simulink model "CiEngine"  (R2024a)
settings: Solver=VariableStepAuto  StartTime=0.0  StopTime=inf  RelTol=1e-3  EnableMultiTasking=on
model workspace (MAT data in the model file):
  AccPwrTbl : Simulink.Parameter (value not decoded)
  AccSpdBpts : Simulink.Parameter (value not decoded)
  TimeCnstECP : Simulink.Parameter (value not decoded)
  TimeCnstEGR : Simulink.Parameter (value not decoded)
  TimeCnstETC : Simulink.Parameter (value not decoded)
  TimeCnstICP : Simulink.Parameter (value not decoded)
  TimeCnstIVL : Simulink.Parameter (value not decoded)
  TimeCnstSWVA : Simulink.Parameter (value not decoded)
  TimeCnstVCR : Simulink.Parameter (value not decoded)
  TimeCnstVGT : Simulink.Parameter (value not decoded)
  TimeCnstVIRL : Simulink.Parameter (value not decoded)
  TimeCnstWGA : Simulink.Parameter (value not decoded)
symbols that are objects in the model workspace (value not decoded): TimeCnstECP, TimeCnstEGR, TimeCnstETC, TimeCnstICP, TimeCnstIVL, TimeCnstSWVA, TimeCnstVCR, TimeCnstVGT, TimeCnstVIRL, TimeCnstWGA
libraries: autolibhevctrlrcommon x1, autolibpowerinfoutils x1, autolibutils x1

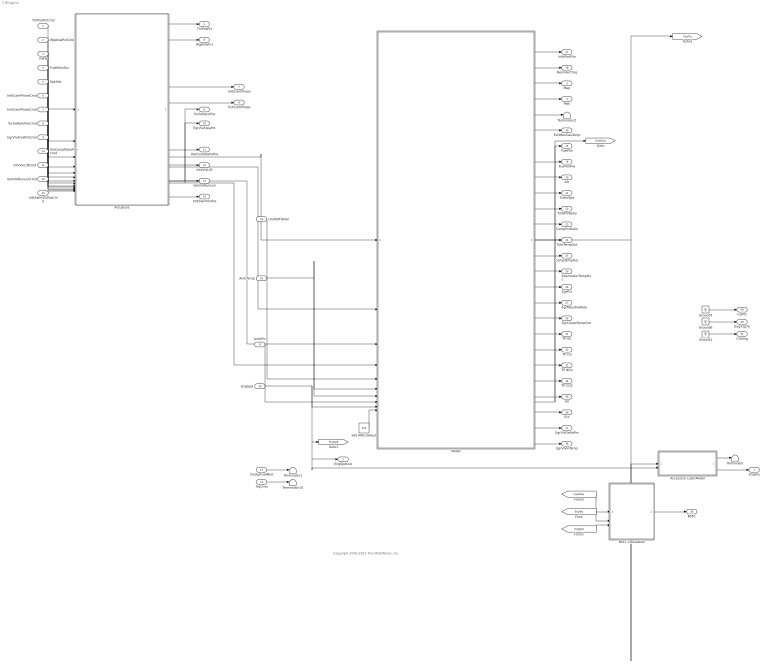
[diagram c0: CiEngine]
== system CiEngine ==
  note: Copyright 2020-2021 The MathWorks, Inc.
  ThrPosPctCmd : Inport
  WgAreaPctCmd : Inport  Port=2
  InjPw : Inport  Port=3
  FuelMainSoi : Inport  Port=4
  SpkAdv : Inport  Port=5
  IntkCamPhaseCmd : Inport  Port=6
  ExhCamPhaseCmd : Inport  Port=7
  TurboRackPosCmd : Inport  Port=8
  EgrVlvAreaPctCmd : Inport  Port=9
  VarCompRatioPosCmd : Inport  Port=10
  IntkVlvLiftCmd : Inport  Port=11
  VarIntkRunLenCmd : Inport  Port=12
  ClsdLpFuelMult : Inport  Port=13  Unit=1
  IntkSwirlVlvPosCmd : Inport  Port=14
  TrqCmd : Inport  Port=15  Unit=N*m
  AmbTemp : Inport  Port=16
  AmbPrs : Inport  Port=17
  EngSpd : Inport  Port=18  Interpolate=off
  UndHdFlwVel : Inport  Port=19
  100 MPa Default : Constant  Value=100
  Accessory Load Model : Subsystem
  Actuators : Subsystem
  BSFC Calculation : Subsystem
  Ground1 : Ground
  Ground5 : Ground
  Ground6 : Ground
  Model : ModelReference  ModelNameDialog=CiEngineCore  SimulationMode=Normal  ModelReferenceVersion=8.0
  Terminator{,1..2,15} (4 alike) : Terminator
  EngTrq : Outport  Unit=N*m  VectorParamsAs1DForOutWhenUnconnected=off
  EngSpdOut : Outport  Port=2  VectorParamsAs1DForOutWhenUnconnected=off
  Map : Outport  Port=3  VectorParamsAs1DForOutWhenUnconnected=off
  Mat : Outport  Port=4  VectorParamsAs1DForOutWhenUnconnected=off
  ThrPosPct : Outport  Port=5  VectorParamsAs1DForOutWhenUnconnected=off
  WgAreaPct : Outport  Port=6  VectorParamsAs1DForOutWhenUnconnected=off
  IntkCamPhase : Outport  Port=7  VectorParamsAs1DForOutWhenUnconnected=off
  ExhCamPhase : Outport  Port=8  VectorParamsAs1DForOutWhenUnconnected=off
  TurboRackPos : Outport  Port=9  VectorParamsAs1DForOutWhenUnconnected=off
  EgrVlvAreaPct : Outport  Port=10  VectorParamsAs1DForOutWhenUnconnected=off
  VarCompRatioPos : Outport  Port=11  VectorParamsAs1DForOutWhenUnconnected=off
  IntkVlvLift : Outport  Port=12  VectorParamsAs1DForOutWhenUnconnected=off
  VarIntkRunLen : Outport  Port=13  VectorParamsAs1DForOutWhenUnconnected=off
  IntkSwirlVlvPos : Outport  Port=14  VectorParamsAs1DForOutWhenUnconnected=off
  FuelFlw : Outport  Port=15  VectorParamsAs1DForOutWhenUnconnected=off
  FuelVolFlw : Outport  Port=16  VectorParamsAs1DForOutWhenUnconnected=off
  IntkPortFlw : Outport  Port=17  VectorParamsAs1DForOutWhenUnconnected=off
  NormAirChrg : Outport  Port=18  VectorParamsAs1DForOutWhenUnconnected=off
  ExhManGasTemp : Outport  Port=19  VectorParamsAs1DForOutWhenUnconnected=off
  Afr : Outport  Port=20  VectorParamsAs1DForOutWhenUnconnected=off
  TurboSpd : Outport  Port=21  VectorParamsAs1DForOutWhenUnconnected=off
  TurbPrsRatio : Outport  Port=22  VectorParamsAs1DForOutWhenUnconnected=off
  CompPrsRatio : Outport  Port=23  VectorParamsAs1DForOutWhenUnconnected=off
  TurbTempOut : Outport  Port=24  VectorParamsAs1DForOutWhenUnconnected=off
  CompTempOut : Outport  Port=25  VectorParamsAs1DForOutWhenUnconnected=off
  EgrPct : Outport  Port=26  VectorParamsAs1DForOutWhenUnconnected=off
  EgrMassFlwRate : Outport  Port=27  VectorParamsAs1DForOutWhenUnconnected=off
  EgrCoolerTempOut : Outport  Port=28  VectorParamsAs1DForOutWhenUnconnected=off
  IntercoolerTempOut : Outport  Port=29  VectorParamsAs1DForOutWhenUnconnected=off
  BSFC : Outport  Port=30  Unit=g/(kW*hr)  VectorParamsAs1DForOutWhenUnconnected=off
  TP HC : Outport  Port=31  VectorParamsAs1DForOutWhenUnconnected=off
  TP CO : Outport  Port=32  VectorParamsAs1DForOutWhenUnconnected=off
  TP NOx : Outport  Port=33  VectorParamsAs1DForOutWhenUnconnected=off
  TP CO2 : Outport  Port=34  VectorParamsAs1DForOutWhenUnconnected=off
  Iat : Outport  Port=35  VectorParamsAs1DForOutWhenUnconnected=off
  Ect : Outport  Port=36  VectorParamsAs1DForOutWhenUnconnected=off
  EgrVlvDeltaPrs : Outport  Port=37  VectorParamsAs1DForOutWhenUnconnected=off
  EgrVlvInTemp : Outport  Port=38  VectorParamsAs1DForOutWhenUnconnected=off
  CylPrs : Outport  Port=39  VectorParamsAs1DForOutWhenUnconnected=off
  EngTrqCrk : Outport  Port=40  VectorParamsAs1DForOutWhenUnconnected=off
  CrkAng : Outport  Port=41  VectorParamsAs1DForOutWhenUnconnected=off
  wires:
  EngSpd/1 -> Accessory Load Model/2(EngSpd), EngSpdOut/1, [EngSpd], Model/9
  Model/1 -> Accessory Load Model/1(EngTrqIn), [EngTrq]
  TrqCmd/1 -> Terminator15/1
  [FuelFlow] -> BSFC Calculation/1(FuelFlow)
  [EngTrq] -> BSFC Calculation/2(EngTrq)
  [EngSpd] -> BSFC Calculation/3(EngSpd)
  BSFC Calculation/1(BSFC (g/Kwh)) -> BSFC/1
  Model/8 -> FuelFlw/1, [FuelFlow]
  AmbTemp/1 -> Model/6, Model/7
  Actuators/1(ThrPosPct) -> ThrPosPct/1
  Actuators/2(WgAreaPct) -> WgAreaPct/1
  AmbPrs/1 -> Model/8
  UndHdFlwVel/1 -> Model/5
  Actuators/3(InjPw) -> Model/1
  Actuators/4(FuelMainSoi) -> Model/2
  Actuators/7(TurboRackPos) -> TurboRackPos/1, Model/3
  Actuators/8(EgrVlvAreaPct) -> EgrVlvAreaPct/1, Model/4
  Actuators/5(IntkCamPhase) -> IntkCamPhase/1
  Actuators/6(ExhCamPhase) -> ExhCamPhase/1
  Actuators/9(VarCompRatioPos) -> VarCompRatioPos/1
  Actuators/10(IntkVlvLift) -> IntkVlvLift/1
  Actuators/12(IntkSwirlVlvPos) -> IntkSwirlVlvPos/1
  Actuators/11(VarIntkRunLen) -> VarIntkRunLen/1
  ThrPosPctCmd/1 -> Actuators/1(ThrPosPctCmd)
  WgAreaPctCmd/1 -> Actuators/2(WgAreaPctCmd)
  InjPw/1 -> Actuators/3(InjPwCmd)
  FuelMainSoi/1 -> Actuators/4(FuelMainSoiCmd)
  SpkAdv/1 -> Actuators/5(SpkAdvCmd)
  IntkCamPhaseCmd/1 -> Actuators/6(IntkCamPhaseCmd)
  ExhCamPhaseCmd/1 -> Actuators/7(ExhCamPhaseCmd)
  TurboRackPosCmd/1 -> Actuators/8(TurboRackPosCmd)
  EgrVlvAreaPctCmd/1 -> Actuators/9(EgrVlvAreaPctCmd)
  VarCompRatioPosCmd/1 -> Actuators/10(VarCompRatioPosCmd)
  IntkVlvLiftCmd/1 -> Actuators/11(IntkVlvLiftCmd)
  VarIntkRunLenCmd/1 -> Actuators/12(VarIntkRunLenCmd)
  ClsdLpFuelMult/1 -> Terminator1/1
  IntkSwirlVlvPosCmd/1 -> Actuators/13(IntkSwirlVlvPosCmd)
  Model/2 -> IntkPortFlw/1
  Model/3 -> NormAirChrg/1
  Model/4 -> Map/1
  Model/5 -> Mat/1
  Model/7 -> ExhManGasTemp/1
  Model/6 -> Terminator2/1
  Model/10 -> Afr/1
  Model/11 -> TurboSpd/1
  Model/12 -> TurbPrsRatio/1
  Model/13 -> CompPrsRatio/1
  Model/14 -> TurbTempOut/1
  Model/15 -> CompTempOut/1
  Model/16 -> IntercoolerTempOut/1
  Model/17 -> EgrPct/1
  Model/18 -> EgrMassFlwRate/1
  Model/19 -> EgrCoolerTempOut/1
  Model/20 -> TP HC/1
  Model/21 -> TP CO/1
  Model/22 -> TP NOx/1
  Model/23 -> TP CO2/1
  Model/25 -> Ect/1
  Model/26 -> EgrVlvDeltaPrs/1
  Model/27 -> EgrVlvInTemp/1
  Model/24 -> Iat/1
  100 MPa Default/1 -> Model/10
  Accessory Load Model/2(EngTrqOut) -> EngTrq/1
  Accessory Load Model/1(PwrInfo) -> Terminator/1
  Model/9 -> FuelVolFlw/1
  Ground5/1 -> CylPrs/1
  Ground6/1 -> EngTrqCrk/1
  Ground1/1 -> CrkAng/1

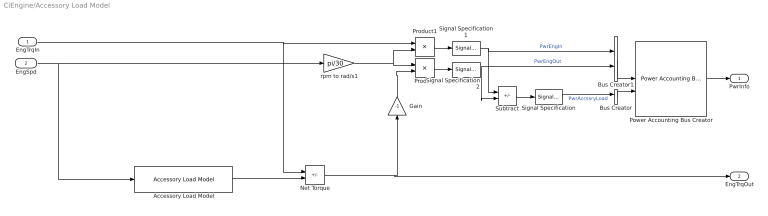
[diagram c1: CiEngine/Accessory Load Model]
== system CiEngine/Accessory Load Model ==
  EngTrqIn : Inport
  EngSpd : Inport  Port=2
  Accessory Load Model : autolibhevctrlrcommon/Accessory Load Model  AccPwrTbl=AccPwrTbl  AccSpdBpts=AccSpdBpts
  Bus Creator : BusCreator  Inputs=1
  Bus Creator1 : BusCreator  Inputs=2
  Gain : Gain  Gain=-1
  Net Torque : Sum  Inputs=+-
  Power Accounting Bus Creator : autolibpowerinfoutils/Power Accounting Bus Creator  AssctBlkSelPopup=Parent  RefBlkName='libraryname/blkname'  PwrTrnsfrdCheckBox=on  PwrNotTrnsfrdCheckBox=on  PwrStoredCheckBox=off  aMode=aMode
  Product : Product
  Product1 : Product
  Signal Specification : SignalSpecification  Unit=W
  Signal Specification1 : SignalSpecification  Unit=W
  Signal Specification2 : SignalSpecification  Unit=W
  Subtract : Sum  Inputs=--
  rpm to rad/s1 : Gain  Gain=pi/30
  PwrInfo : Outport  VectorParamsAs1DForOutWhenUnconnected=off
  EngTrqOut : Outport  Port=2  Unit=N*m  VectorParamsAs1DForOutWhenUnconnected=off
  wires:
  EngSpd/1 -> Accessory Load Model/1, rpm to rad/s1/1
  Net Torque/1 -> EngTrqOut/1, Gain/1
  Bus Creator/1 -> Power Accounting Bus Creator/2
  Bus Creator1/1 -> Power Accounting Bus Creator/1
  EngTrqIn/1 -> Product1/1, Net Torque/1
  Subtract/1 -> Signal Specification/1
  Signal Specification/1 -> Bus Creator/1  "PwrAccssryLoad"
  Power Accounting Bus Creator/1 -> PwrInfo/1
  Product/1 -> Signal Specification2/1
  Product1/1 -> Signal Specification1/1
  rpm to rad/s1/1 -> Product1/2, Product/1
  Signal Specification1/1 -> Subtract/1, Bus Creator1/1  "PwrEngIn"
  Signal Specification2/1 -> Subtract/2, Bus Creator1/2  "PwrEngOut"
  Gain/1 -> Product/2
  Accessory Load Model/1 -> Net Torque/2

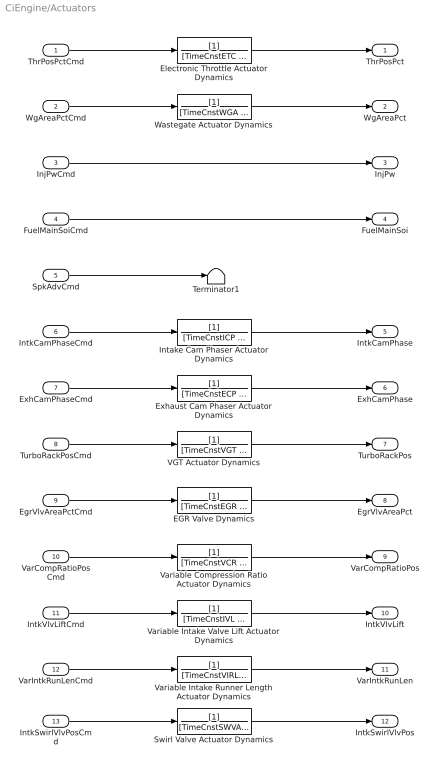
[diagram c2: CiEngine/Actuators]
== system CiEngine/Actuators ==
  ThrPosPctCmd : Inport  Unit=%
  WgAreaPctCmd : Inport  Port=2  Unit=%
  InjPwCmd : Inport  Port=3  Unit=ms
  FuelMainSoiCmd : Inport  Port=4  Unit=deg
  SpkAdvCmd : Inport  Port=5  Unit=deg
  IntkCamPhaseCmd : Inport  Port=6  Unit=deg
  ExhCamPhaseCmd : Inport  Port=7  Unit=deg
  TurboRackPosCmd : Inport  Port=8  Unit=1
  EgrVlvAreaPctCmd : Inport  Port=9  Unit=%
  VarCompRatioPosCmd : Inport  Port=10
  IntkVlvLiftCmd : Inport  Port=11
  VarIntkRunLenCmd : Inport  Port=12
  IntkSwirlVlvPosCmd : Inport  Port=13
  EGR Valve Dynamics : TransferFcn  Denominator=[TimeCnstEGR 1]
  Electronic Throttle Actuator Dynamics : TransferFcn  Denominator=[TimeCnstETC 1]
  Exhaust Cam Phaser Actuator Dynamics : TransferFcn  Denominator=[TimeCnstECP 1]
  Intake Cam Phaser Actuator Dynamics : TransferFcn  Denominator=[TimeCnstICP 1]
  Swirl Valve Actuator Dynamics : TransferFcn  Denominator=[TimeCnstSWVA 1]
  Terminator1 : Terminator
  VGT Actuator Dynamics : TransferFcn  Denominator=[TimeCnstVGT 1]
  Variable Compression Ratio Actuator Dynamics : TransferFcn  Denominator=[TimeCnstVCR 1]
  Variable Intake Runner Length Actuator Dynamics : TransferFcn  Denominator=[TimeCnstVIRL 1]
  Variable Intake Valve Lift Actuator Dynamics : TransferFcn  Denominator=[TimeCnstIVL 1]
  Wastegate Actuator Dynamics : TransferFcn  Denominator=[TimeCnstWGA 1]
  ThrPosPct : Outport  Unit=%  VectorParamsAs1DForOutWhenUnconnected=off
  WgAreaPct : Outport  Port=2  Unit=%  VectorParamsAs1DForOutWhenUnconnected=off
  InjPw : Outport  Port=3  VectorParamsAs1DForOutWhenUnconnected=off
  FuelMainSoi : Outport  Port=4  VectorParamsAs1DForOutWhenUnconnected=off
  IntkCamPhase : Outport  Port=5  Unit=deg  VectorParamsAs1DForOutWhenUnconnected=off
  ExhCamPhase : Outport  Port=6  Unit=deg  VectorParamsAs1DForOutWhenUnconnected=off
  TurboRackPos : Outport  Port=7  Unit=1  VectorParamsAs1DForOutWhenUnconnected=off
  EgrVlvAreaPct : Outport  Port=8  Unit=%  VectorParamsAs1DForOutWhenUnconnected=off
  VarCompRatioPos : Outport  Port=9  VectorParamsAs1DForOutWhenUnconnected=off
  IntkVlvLift : Outport  Port=10  VectorParamsAs1DForOutWhenUnconnected=off
  VarIntkRunLen : Outport  Port=11  VectorParamsAs1DForOutWhenUnconnected=off
  IntkSwirlVlvPos : Outport  Port=12  VectorParamsAs1DForOutWhenUnconnected=off
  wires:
  Variable Compression Ratio Actuator Dynamics/1 -> VarCompRatioPos/1
  Variable Intake Valve Lift Actuator Dynamics/1 -> IntkVlvLift/1
  Variable Intake Runner Length Actuator Dynamics/1 -> VarIntkRunLen/1
  Swirl Valve Actuator Dynamics/1 -> IntkSwirlVlvPos/1
  Intake Cam Phaser Actuator Dynamics/1 -> IntkCamPhase/1
  Exhaust Cam Phaser Actuator Dynamics/1 -> ExhCamPhase/1
  Wastegate Actuator Dynamics/1 -> WgAreaPct/1
  Electronic Throttle Actuator Dynamics/1 -> ThrPosPct/1
  FuelMainSoiCmd/1 -> FuelMainSoi/1
  IntkVlvLiftCmd/1 -> Variable Intake Valve Lift Actuator Dynamics/1
  IntkSwirlVlvPosCmd/1 -> Swirl Valve Actuator Dynamics/1
  WgAreaPctCmd/1 -> Wastegate Actuator Dynamics/1
  ThrPosPctCmd/1 -> Electronic Throttle Actuator Dynamics/1
  ExhCamPhaseCmd/1 -> Exhaust Cam Phaser Actuator Dynamics/1
  IntkCamPhaseCmd/1 -> Intake Cam Phaser Actuator Dynamics/1
  VarCompRatioPosCmd/1 -> Variable Compression Ratio Actuator Dynamics/1
  VarIntkRunLenCmd/1 -> Variable Intake Runner Length Actuator Dynamics/1
  InjPwCmd/1 -> InjPw/1
  VGT Actuator Dynamics/1 -> TurboRackPos/1
  EGR Valve Dynamics/1 -> EgrVlvAreaPct/1
  TurboRackPosCmd/1 -> VGT Actuator Dynamics/1
  EgrVlvAreaPctCmd/1 -> EGR Valve Dynamics/1
  SpkAdvCmd/1 -> Terminator1/1

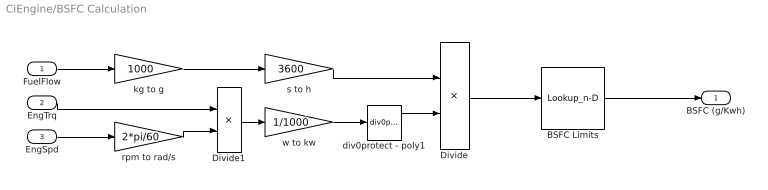
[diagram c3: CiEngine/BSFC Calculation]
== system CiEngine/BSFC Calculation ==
  FuelFlow : Inport
  EngTrq : Inport  Port=2
  EngSpd : Inport  Port=3
  BSFC Limits : Lookup_n-D  NumberOfTableDimensions=1  BreakpointsForDimension1=[0 500]  Table=[0 500]  ExtrapMethod=Clip  InternalRulePriority=Speed  RndMeth=Simplest
  Divide : Product  Inputs=*/
  Divide1 : Product  Inputs=**
  div0protect - poly1 : autolibutils/div0protect - poly  thresh=1e-6  ZeroCross1=off  aMode=aMode
  kg to g : Gain  Gain=1000
  rpm to rad/s : Gain  Gain=2*pi/60
  s to h : Gain  Gain=3600
  w to kw : Gain  Gain=1/1000
  BSFC (g/Kwh) : Outport  VectorParamsAs1DForOutWhenUnconnected=off
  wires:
  Divide1/1 -> w to kw/1
  kg to g/1 -> s to h/1
  FuelFlow/1 -> kg to g/1
  rpm to rad/s/1 -> Divide1/2
  EngSpd/1 -> rpm to rad/s/1
  EngTrq/1 -> Divide1/1
  Divide/1 -> BSFC Limits/1
  w to kw/1 -> div0protect - poly1/1
  s to h/1 -> Divide/1
  BSFC Limits/1 -> BSFC (g/Kwh)/1
  div0protect - poly1/1 -> Divide/2
